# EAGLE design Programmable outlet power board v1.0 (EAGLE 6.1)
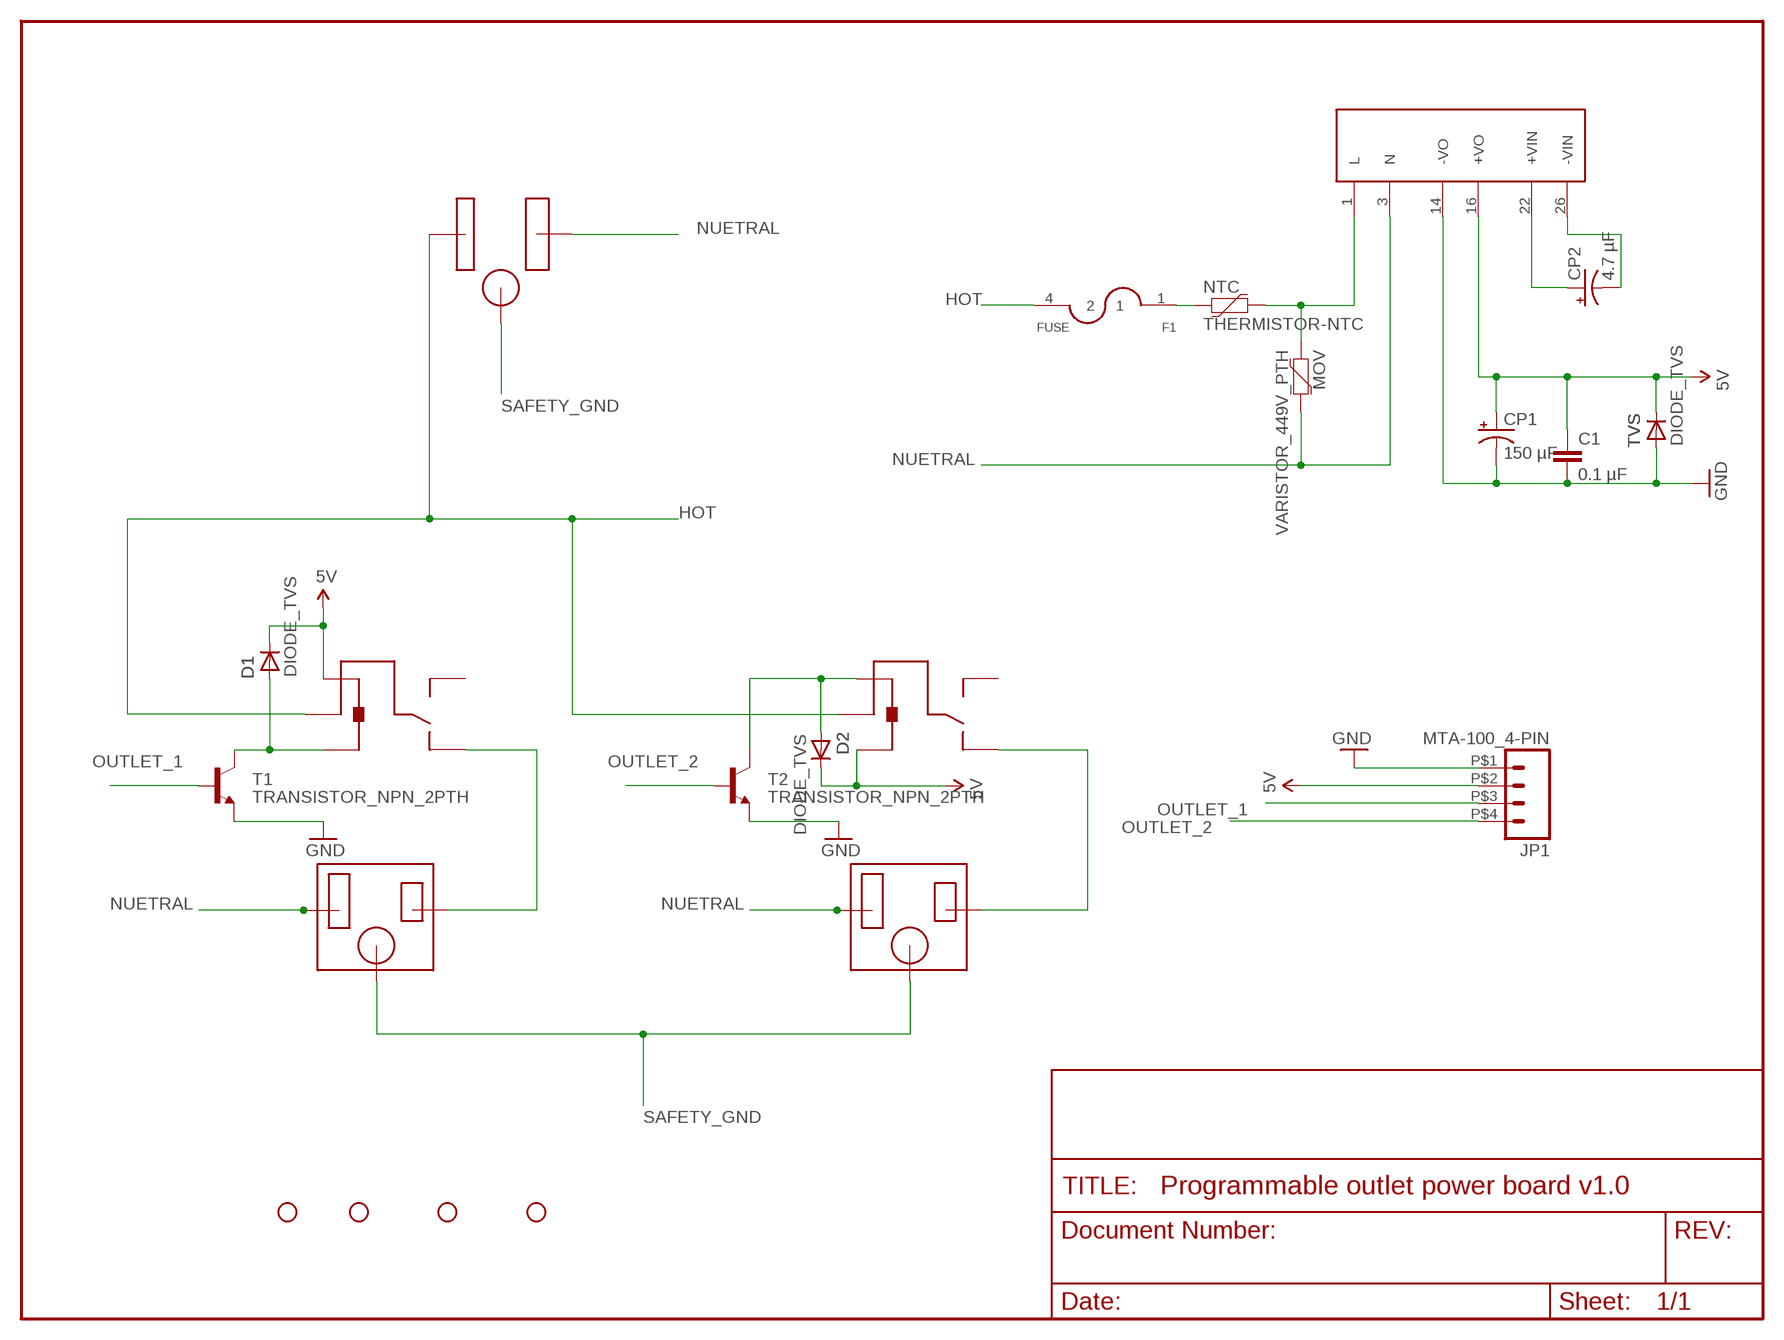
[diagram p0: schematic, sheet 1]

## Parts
AC_DC  VSK-S3-5U  [VSK-S3]
C1  0.1 µF  CAP_PTH_5MM  [CAP_PTH_5MM]
CP1  150 µF  CAP_100UF_50V  [CAP_200_SERIES]
CP2  4.7 µF  CAP_POLPTH4  [CPOL-RADIAL-1000UF-25V]
D1  DIODE_TVS  [DO-41_AXIAL_PTH]
D2  DIODE_TVS  [DO-41_AXIAL_PTH]
F1  FUSE  [FUSE_5X20MM]
JP1  MTA-100_4-PIN  [MTA-100_4-PIN_PCB]
JP2  STAND-OFF  [STAND-OFF]
JP3  STAND-OFF  [STAND-OFF]
JP4  STAND-OFF  [STAND-OFF]
JP5  STAND-OFF  [STAND-OFF]
MOV  VARISTOR_449V_PTH  [DISC_5MM]
NTC  THERMISTOR-NTC  [DISC_3.5MM]
PLUG  OUTLET_PLUG  [OUTLET_PLUG]
RELAY_1  RELAY_G5LE-1A  [SPDT_RELAY]
RELAY_2  RELAY_G5LE-1A  [SPDT_RELAY]
SOCKET_1  OUTLET_RECEPTACLE  [OUTLET_RECEPTACLE]
SOCKET_2  OUTLET_RECEPTACLE  [OUTLET_RECEPTACLE]
T1  TRANSISTOR_NPN_2PTH  [TO-92]
T2  TRANSISTOR_NPN_2PTH  [TO-92]
TVS  DIODE_TVS  [DO-41_AXIAL_PTH]

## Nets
5V: AC_DC.16(+VO) C1.1 CP1.+ D1.CATHODE(C) D2.CATHODE(C) JP1.P$2 RELAY_1.PIN_2 RELAY_2.PIN_5 TVS.CATHODE(C)
GND: AC_DC.14(-VO) C1.2 CP1.- JP1.P$1 T1.3(E) T2.3(E) TVS.ANODE(A)
HOT: F1.4 PLUG.HOT RELAY_1.PIN_1 RELAY_2.PIN_1
N$1: D2.ANODE(A) RELAY_2.PIN_2 T2.1(C)
N$3: RELAY_2.PIN_4_NC SOCKET_2.HOT
N$4: RELAY_1.PIN_4_NC SOCKET_1.HOT
N$5: AC_DC.22(+VIN) CP2.1(+)
N$6: AC_DC.26(-VIN) CP2.2(-)
N$7: F1.1 NTC.P$1
N$8: AC_DC.1(L) MOV.P$1 NTC.P$2
N$9: D1.ANODE(A) RELAY_1.PIN_5 T1.1(C)
NUETRAL: AC_DC.3(N) MOV.P$2 PLUG.NEUTRAL(NUETRAL) SOCKET_1.NUETRAL SOCKET_2.NUETRAL
OUTLET_1: JP1.P$3 T1.2(B)
OUTLET_2: JP1.P$4 T2.2(B)
SAFETY_GND: PLUG.GND SOCKET_1.GND SOCKET_2.GND
Unconnected: RELAY_1.PIN_3_NO RELAY_2.PIN_3_NO

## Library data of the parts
AC_DC = Misc:VSK-S3-5U
C1 = Capacitors:CAP_PTH_5MM
CP1 = Capacitors:CAP_100UF_50V
CP2 = SparkFun:CAP_POL: Capacitor Polarized
D1 D2 TVS = Diodes:DIODE_TVS
F1 = Misc:FUSE
JP1 = Connectors:MTA-100_4-PIN
JP2-JP5 = SparkFun-Electromechanical:STAND-OFF: #4 Stand Off
MOV = Diodes:VARISTOR_449V_PTH: Digi-Key F3361-ND
NTC = Diodes:THERMISTOR-NTC
PLUG = Misc:OUTLET_PLUG
RELAY_1 RELAY_2 = Misc:RELAY_G5LE-1A
SOCKET_1 SOCKET_2 = Misc:OUTLET_RECEPTACLE
T1 T2 = SparkFun:TRANSISTOR_NPN_2

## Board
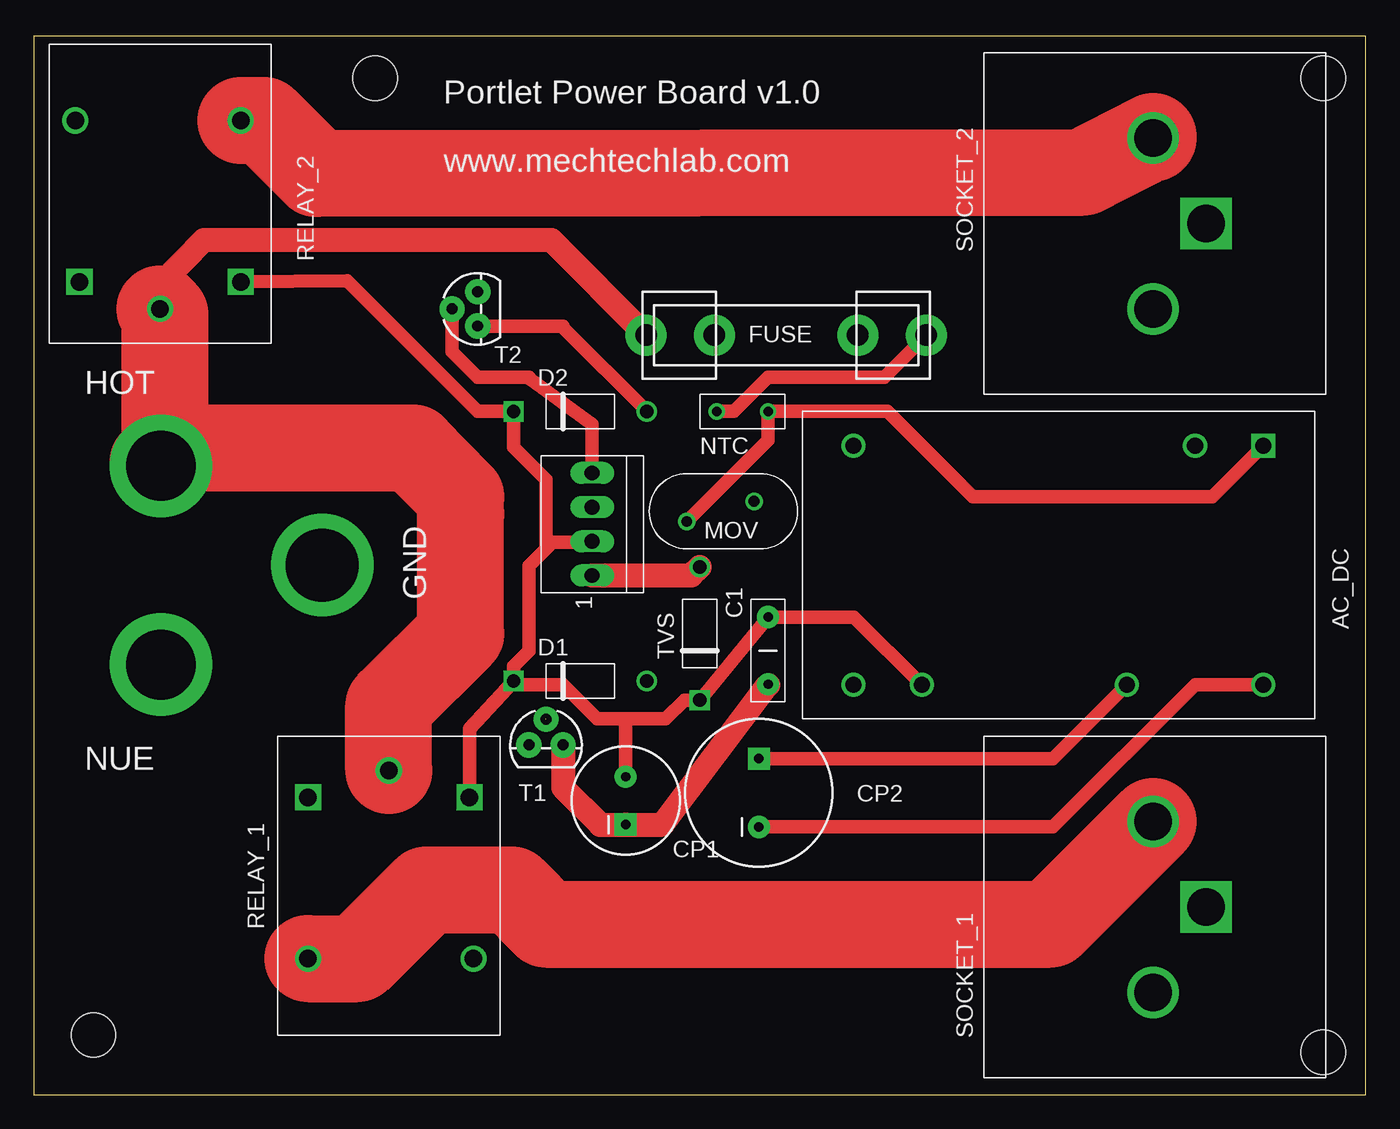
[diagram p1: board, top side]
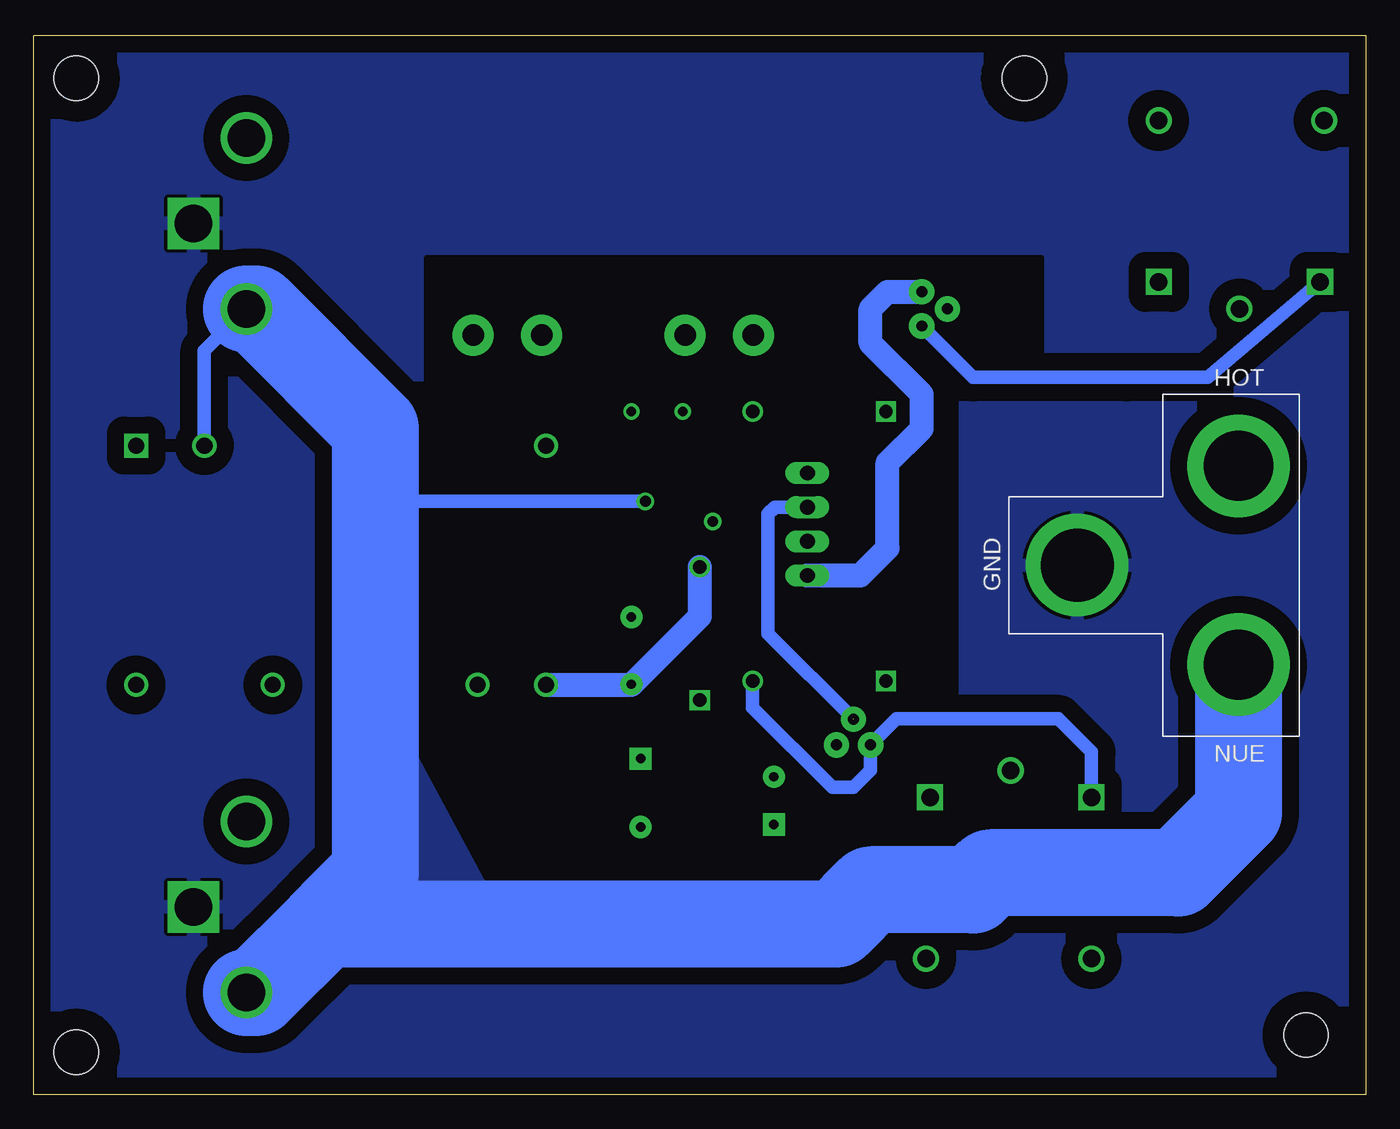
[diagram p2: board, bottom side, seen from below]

Size 99.06 x 78.74 mm. Coordinates in mm from the lower left corner, seen from the top.
Outline: 0,0 99.06,0 99.06,78.74 0,78.74 0,0
Copper layers (1*16): Top 0.035mm / dielectric 1.5mm / Bottom 0.035mm
Design rules: minimum track width 25mil, minimum drill 24mil, track to track 30mil, track to pad 20mil, pad to pad 20mil, via to via 8mil, smd to smd 8mil, copper to edge 40mil, drill to drill 8mil, minimum pad ring 10mil, minimum via ring 8mil, stop-mask expansion 4mil, vias tented up to drill 0mil, thermal gap 10mil

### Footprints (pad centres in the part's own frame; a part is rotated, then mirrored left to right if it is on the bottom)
VSK-S3 = drill 1.2 square: 1 0,0 | drill 1.2: 3 5.08,0; 13 30.48,0; 14 30.48,17.78; 16 25.4,17.78; 22 10.16,17.78; 26 0,17.78
CAP_PTH_5MM = drill 0.7 pad 1.651: 1 -2.5,0; 2 2.5,0
CAP_200_SERIES = drill 0.7 pad 1.651: + 3.556,0 | drill 0.7 pad 1.651 square: - 0,0
CPOL-RADIAL-1000UF-25V = drill 0.7 pad 1.651 square: 1 2.54,0 | drill 0.7 pad 1.651: 2 -2.54,0
DO-41_AXIAL_PTH = drill 1: ANODE 4.953,0 | drill 1 square: CATHODE -4.953,0
FUSE_5X20MM = drill 1.6 pad 3.048: 1 0,-10.414; 2 0,-5.334; 3 0,5.334; 4 0,10.414
MTA-100_4-PIN_PCB = drill 1.1 long: P$1 0,0; P$2 2.54,0; P$3 5.08,0; P$4 7.62,0
STAND-OFF = hole 3.302: 0,0
DISC_5MM = drill 0.8: P$1 0,0; P$2 5.004,1.499
DISC_3.5MM = drill 0.7: P$1 -1.27,0; P$2 2.54,0
OUTLET_PLUG = drill 5.41 pad 7.62: GND 0,0 | drill 5.182 pad 7.62: HOT -7.391,11.989; NEUTRAL 7.391,11.989
SPDT_RELAY = drill 1.3: PIN_1 0.01,-0.005; PIN_3_NO 14.01,6.295; PIN_4_NC 14.01,-6.005 | drill 1.3 square: PIN_2 2.01,5.995; PIN_5 2.01,-6.005
OUTLET_RECEPTACLE = drill 2.8 square: GND 0,0 | drill 2.8: HOT 6.35,3.937; NUETRAL -6.35,3.937
TO-92 = drill 0.813 pad 1.88: 1 -1.27,0; 2 0,1.905; 3 1.27,0

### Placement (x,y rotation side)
AC_DC  91.44,48.26 180 top
C1  54.61,33.02 270 top
CP1  44.02,20.09 90 top
CP2  53.92,22.45 90 top
D1  40.64,30.76 0 top
D2  40.64,50.8 0 top
F1  55.96,56.46 90 top
JP1  41.53,38.61 90 top
JP2  4.45,4.45 0 top
JP3  25.4,75.56 0 top
JP4  95.89,75.56 0 top
JP5  95.89,3.17 0 top
MOV  48.56,42.62 0 top
NTC  52.07,50.8 0 top
PLUG  21.46,39.37 270 bottom
RELAY_1  26.42,24.13 270 top
RELAY_2  9.4,58.42 90 top
SOCKET_1  87.17,13.97 90 top
SOCKET_2  87.17,64.77 90 top
T1  38.1,26.01 0 top
T2  33.02,58.42 90 top
TVS  49.53,34.29 90 top

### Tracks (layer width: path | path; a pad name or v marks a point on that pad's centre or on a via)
5V
  Top 1.016: AC_DC.16 61,35.52 C1.1 54.61,35.56 54.3,35.13 TVS.CATHODE 48.39,29.34 46.99,27.94 43.97,27.94 | D1.CATHODE 35.69,31.88 36.83,33.02 36.83,39.32 38.12,40.62 | 38.12,40.62 38.58,41.07 41.45,41.07 JP1.P$2 | RELAY_2.PIN_5 23.31,60.51 33.02,50.8 D2.CATHODE 35.69,48.13 38.1,45.72 38.1,40.64 38.12,40.62 | RELAY_1.PIN_2 32.41,27.2 D1.CATHODE | 43.97,23.65 44.04,23.57 44.09,23.57 CP1.+ 44.02,27.89 43.97,27.94 | 43.97,27.94 41.91,27.94 39.37,30.48 35.56,30.48 35.69,30.61 D1.CATHODE
GND
  Top 1.016: 54.61,30.48 C1.2 | 43.99,20.07 CP1.-
  Top 1.778: JP1.P$1 48.9,38.61 TVS.ANODE | CP1.- 46.76,20.09 54.61,30.48 | T1.3 39.37,22.84 42.14,20.07 43.99,20.07
  Bottom 1.778: AC_DC.14 54.65,30.48 C1.2 54.57,30.52 49.53,35.56 TVS.ANODE | JP1.P$1 37.59,38.61 35.56,40.64 35.56,46.99 33.02,49.53 33.02,52.07 36.83,55.88 36.83,58.42 35.56,59.69 T2.3
HOT
  Top 1.778: RELAY_2.PIN_1 9.53,60.33 12.68,63.55 38.48,63.55 F1.4
  Top 6.452: RELAY_1.PIN_1 26.41,28.95 26.67,29.21 31.75,34.29 31.75,43.18 31.75,44.45 28.22,48.08 11.25,48.08 PLUG.HOT 9.25,46.99 8.89,46.99 9.75,47.85 9.75,58.01 | 9.75,58.01 9.53,58.24 | RELAY_2.PIN_1 9.51,58.26 9.75,58.01
N$1
  Top 1.016: T2.1 39.37,57.15 39.37,57.02 D2.ANODE
  Bottom 1.016: RELAY_2.PIN_2 11.76,53.34 17.78,53.34 29.21,53.34 T2.1
N$2
  cutout Bottom (isolate 2.54): 22.86,16.51 22.86,22.86 29.21,22.86
N$3
  Top 6.452: RELAY_2.PIN_4_NC 17.11,72.43 21.03,68.5 78.05,68.58 83.24,71.22 SOCKET_2.HOT
N$4
  Top 6.452: RELAY_1.PIN_4_NC 24.09,10.12 29.21,15.24 35.56,15.24 38.1,12.7 75.62,12.7 SOCKET_1.HOT
N$5
  Top 1.016: CP2.1 75.79,24.99 AC_DC.22
N$6
  Top 1.016: CP2.2 75.79,19.91 86.36,30.48 AC_DC.26
N$7
  Top 1.016: NTC.P$1 52.07,50.8 54.61,53.34 63.25,53.34 F1.1
N$8
  Top 1.016: AC_DC.1 87.63,44.45 69.85,44.45 63.5,50.8 NTC.P$2 54.61,48.67 MOV.P$1
N$9
  Bottom 1.016: RELAY_1.PIN_5 20.41,25.49 22.86,27.94 34.9,27.94 T1.1 36.83,24.13 38.1,22.86 39.67,22.86 45.59,28.78 D1.ANODE
N$10
  cutout Bottom: 24.13,62.23 24.13,52.07 30.48,52.07 30.48,17.78 62.23,17.78 62.23,26.67 69.85,26.67 69.85,62.23
NUETRAL
  Bottom 1.016: AC_DC.3 86.36,55.3 SOCKET_2.NUETRAL 74.93,50.11 74.93,45.72 73.33,44.12 MOV.P$2
  Bottom 6.452: SOCKET_2.NUETRAL 82.55,58.42 73.66,49.53 73.66,17.2 | PLUG.NEUTRAL 9.47,21.01 13.97,16.51 27.94,16.51 29.21,15.24 36.83,15.24 39.37,12.7 77.47,12.7 | SOCKET_1.NUETRAL 82.55,7.62 77.47,12.7 | 77.47,12.7 76.2,13.97 | 76.2,13.97 73.66,16.51 | 73.66,16.51 76.2,13.97 | 76.2,13.97 77.47,12.7 | 77.47,12.7 76.2,13.97 | 76.2,13.97 73.66,16.51
  pour Bottom: 73.66,29.21 64.77,12.7 73.66,12.7
OUTLET_1  (1 unrouted)
  Bottom 1.016: JP1.P$3 43.94,43.69 44.45,43.18 44.45,34.29 38.1,27.94
OUTLET_2
  Top 1.016: T2.2 31.11,55.24 33.02,53.34 36.83,53.34 36.83,53.26 41.5,49.86 41.5,46.15 41.5,46.23 JP1.P$4
SAFETY_GND
  pour Bottom (isolate 1.27): 0,78.74 0,0 99.06,0 99.06,78.74

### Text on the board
tPlace: Portlet Power Board v1.0 | www.mechtechlab.com | FUSE | HOT | GND | NUE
